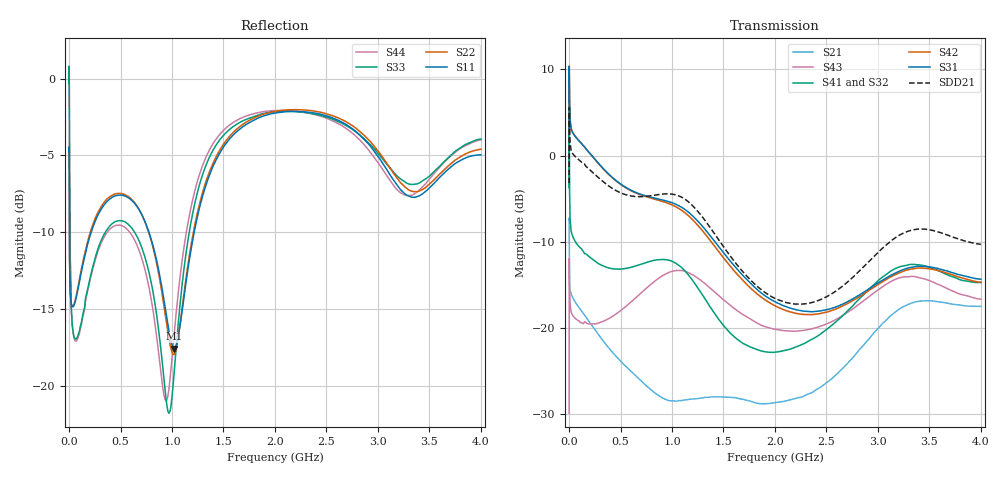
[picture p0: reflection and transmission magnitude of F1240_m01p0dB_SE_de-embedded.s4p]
! Integrated Device Technology
! Corporate Headquarters
! 6024 Silver Creek Valley Road
! San Jose, CA 95138  USA
! Phone:  1-408-284-8200
! Toll Free:  1-800-223-1366
! Webpage:  http://www.idt.com/
! Timing and RF Division
! 515 Groton Road, Suite 102
! Westford, MA 01886-6024
! Device:  F1240
! Description: Dual Intermediate Frequency Digital Variable Gain Amplifier
! Frequency:  10.0 -  500.00 MHz
! Package:  5x5 mm QFN Plastic Package: 32 pin
! Ports:  8 RF, 20 DC
!  Pin  1  = GA3 / Data  Pin 17  = RF OUT_B+
!  Pin  2  = GA4 / CLK  Pin 18  = RF OUT_B-
!  Pin  3  = GA5  Pin 19  = STBY_B
!  Pin  4  = VMODE  Pin 20  = Ground
!  Pin  5  = No Connect  Pin 21  = Ground
!  Pin  6  = GB5  Pin 22  = STB_A
!  Pin  7  = GB4  Pin 23  = RF OUT_A-  = Port 4
!  Pin  8  = GB3  Pin 24  = RF OUT_A+  = Port 3
!  Pin  9  = GB2  Pin 25  = GA0
!  Pin 10  = GB1  Pin 26  = ISET_A
!  Pin 11  = RF IN_B+  Pin 27  = VCC
!  Pin 12  = RF IN_B-  Pin 28  = Ground
!  Pin 13  = Ground  Pin 29  = RF IN_A-  = Port 2
!  Pin 14  = VCC  Pin 30  = RF IN_A+  = Port 1
!  Pin 15  = ISET_B  Pin 31  = GA1
!  Pin 16  = GB0  Pin 32  = GA2 / CSb
! Gain  = +19.5 dB
! State  = 1
! Voltage  = +5.00 V
! Current  = 85.292 mA (one channel only)
! Temperture  =  +25 C
! Test Date  =  2017-10-18
! Board  =  EB4031
! Data:  The device was measured on a custom evaluation board which has
!  individual transmission lines to the RF pins.  Data was collected
!  using a calibrated network analyzer.  The evaluation board was
!  de-embedded using Automatic Fixture Removal.
!  The reference plane is the edge of the package pin.
!  Only Channel A was measured.
!  This data is in single-ended operation.  If your needs are balanced
!  or differential S-parameters then this file needs to be used a
!  linear simulator.
! File Date:  2017-11-10  MJV
! Note:
!  Integrated Device Technology supplies this data as a sample of measured
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# Hz S dB R 100
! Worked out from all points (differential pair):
!   410 points, 500 kHz to 4 GHz, reference 100 ohm
!   strongest paths, dB at 500 kHz, 930 MHz, 1.96 GHz, 2.98 GHz, 4 GHz:
!     S31: 2.6, -5.2, -16.7, -14.9, -14.3
!     S42: 2.6, -5.4, -17.1, -15.1, -14.7
!     S41: -3.7, -12.1, -22.8, -14.8, -14.7
!     S32: -3.7, -12.2, -22.8, -15.1, -15.2
!     S43: -29.9, -13.8, -20.0, -15.8, -16.6
!     S21: -7.5, -28.2, -28.7, -20.3, -17.5
!   taken as a pair (ports 1,2 in; 3,4 out), SDD21 dB: -3.2, -4.4, -16.3, -11.5, -10.3
!   lowest |S11| = -17.6 dB at 1.02 GHz (marker M1), VSWR 1.30, Z = 78 - j8.28 ohm
!   |S11| at or under -10 dB: 3.562 MHz to 215 MHz (211.4 MHz wide, 193 % of centre); 776.1 MHz to 1.215 GHz (439.3 MHz wide, 44.1 % of centre)
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500000  -4.76 -5.6  -7.51 -5.8  -30.14 80.8  -36.86 78.6
        -7.52 -5.8  -4.76 -5.5  -36.82 77.7  -30.15 81.8
        2.55 -107.5  -3.70 -109.5  -0.31 0.8  -29.87 -43.4
        -3.73 -108.4  2.55 -106.4  -29.88 -43.4  -0.32 3.1
2000000  -6.34 -37.3  -9.77 -38.1  -20.43 32.1  -27.94 10.6
         -9.78 -38.1  -6.31 -37.3  -27.88 10.3  -20.42 32.4
         10.30 -173.2  3.59 169.0  -0.01 -46.7  -11.92 -134.9
         3.56 169.3  10.31 -172.9  -11.90 -135.0  -0.05 -46.3
4000000  -10.67 -41.5  -14.15 -31.0  -20.42 10.9  -30.95 -13.8
         -14.16 -31.0  -10.65 -41.8  -30.90 -14.0  -20.42 11.1
         7.29 162.1  -2.34 140.1  -4.44 -79.3  -13.89 179.4
         -2.39 140.3  7.30 162.3  -13.88 179.3  -4.49 -79.2
1.7e8  -11.05 -104.7  -18.83 -54.0  -22.70 -44.1  -35.70 -29.5
       -18.83 -53.9  -10.88 -106.2  -35.76 -29.3  -22.71 -44.3
       0.69 116.4  -11.48 87.0  -14.03 -142.0  -19.48 109.6
       -11.45 86.9  0.70 115.6  -19.44 109.3  -14.16 -141.9
1.02e9  -17.59 -156.7  -28.86 -170.2  -23.16 149.2  -31.24 -167.0
        -28.45 -171.8  -17.97 -153.8  -31.23 -161.6  -23.84 148.2
        -5.56 -92.7  -12.57 171.4  -19.19 -115.1  -13.57 -121.9
        -12.37 167.6  -5.83 -95.4  -13.37 -121.9  -16.71 -108.1
2.86e9  -3.91 97.5  -22.03 -29.2  -25.36 -154.2  -27.57 -137.9
        -21.99 -29.2  -3.65 98.5  -28.39 -125.4  -26.57 -148.9
        -15.86 -66.0  -16.53 -152.3  -3.88 101.9  -17.76 -80.9
        -16.15 -162.9  -16.06 -63.1  -16.84 -78.6  -4.25 94.9
4e9  -4.96 -141.3  -17.51 105.5  -23.83 -40.1  -24.86 -24.2
     -17.47 105.4  -4.59 -139.5  -25.80 -9.0  -25.55 -33.2
     -14.34 44.4  -15.20 -59.4  -3.92 -134.0  -18.24 66.2
     -14.70 -72.7  -14.70 50.4  -16.65 57.7  -3.98 -143.8
